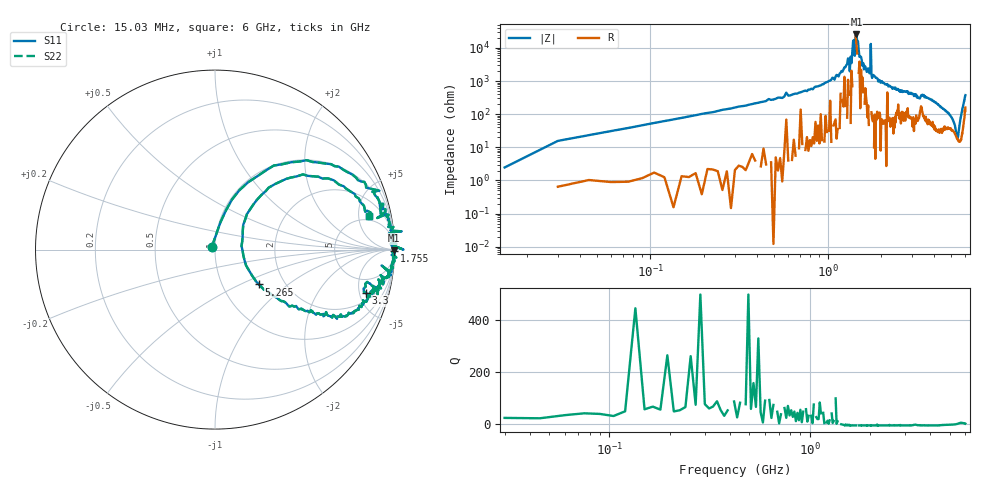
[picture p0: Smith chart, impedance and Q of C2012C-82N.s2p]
!	Network	Analyzer	HP8753E.07.74:	Oct	30	2002	Serial	No.	JP38451487
!	Hewlett-Packard
!	7	Sep	2009	12:10:09
!	Frequency	S11	S21	S12	S22
#	HZ	S	RI	R	50
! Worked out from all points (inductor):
!   400 points, 15.03 MHz to 6 GHz, reference 50 ohm
!   read as one part in series: L = 82.3 nH near 45.03 MHz
!   highest |Z| = 25.5 kohm at 1.455 GHz (marker M1)
!   self-resonance near 1.425 GHz
!   S11 on the Smith chart (normalised r, x): 15.03 MHz: 0.97, +0.03; 1.755 GHz: open; 3.3 GHz: 2.82, -5.76; 5.265 GHz: 1.48, -0.64; 6 GHz: 4.19, +6.79
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1.502992e7  -0.0173 0.0169  1.02 -0.0169  1.02 -0.0169  -0.0173 0.0169
4.502978e7  0.0607 0.218  0.939 -0.218  0.939 -0.218  0.0607 0.218
1.650292e8  0.425 0.487  0.575 -0.487  0.575 -0.487  0.425 0.487
1.020025e9  0.988 0.0963  0.0124 -0.0963  0.0124 -0.0963  0.988 0.0963
1.305023e9  0.995 0.02  0.0051 -0.02  0.0051 -0.02  0.995 0.02
1.335023e9  1.05 6.1e-05  -0.0531 -6.1e-05  -0.0531 -6.1e-05  1.05 6.1e-05
1.395023e9  1 0.00482  -0.00372 -0.00482  -0.00372 -0.00482  1 0.00482
1.425023e9  1 0.0172  -0.0014 -0.0172  -0.0014 -0.0172  1 0.0172
1.455023e9  0.998 -0.00327  0.00214 0.00327  0.00214 0.00327  0.998 -0.00327
1.665022e9  0.992 -0.0518  0.00839 0.0518  0.00839 0.0518  0.992 -0.0518
1.740021e9  0.994 -0.0568  0.0058 0.0568  0.0058 0.0568  0.994 -0.0568
1.755021e9  1 -0.00751  -0.00067 0.00751  -0.00067 0.00751  1 -0.00751
1.770021e9  0.992 -0.0615  0.00827 0.0615  0.00827 0.0615  0.992 -0.0615
1.785021e9  0.989 -0.0787  0.0109 0.0787  0.0109 0.0787  0.989 -0.0787
2.01002e9  0.983 -0.0991  0.0173 0.0991  0.0173 0.0991  0.983 -0.0991
3.015015e9  0.925 -0.216  0.0746 0.216  0.0746 0.216  0.925 -0.216
3.300014e9  0.84 -0.241  0.16 0.241  0.16 0.241  0.84 -0.241
4.00501e9  0.816 -0.32  0.184 0.32  0.184 0.32  0.816 -0.32
5.010005e9  0.426 -0.314  0.574 0.314  0.574 0.314  0.426 -0.314
5.265004e9  0.245 -0.194  0.755 0.194  0.755 0.194  0.245 -0.194
5.415003e9  0.148 0.0196  0.852 -0.0196  0.852 -0.0196  0.148 0.0196
6e9  0.858 0.186  0.142 -0.186  0.142 -0.186  0.858 0.186
